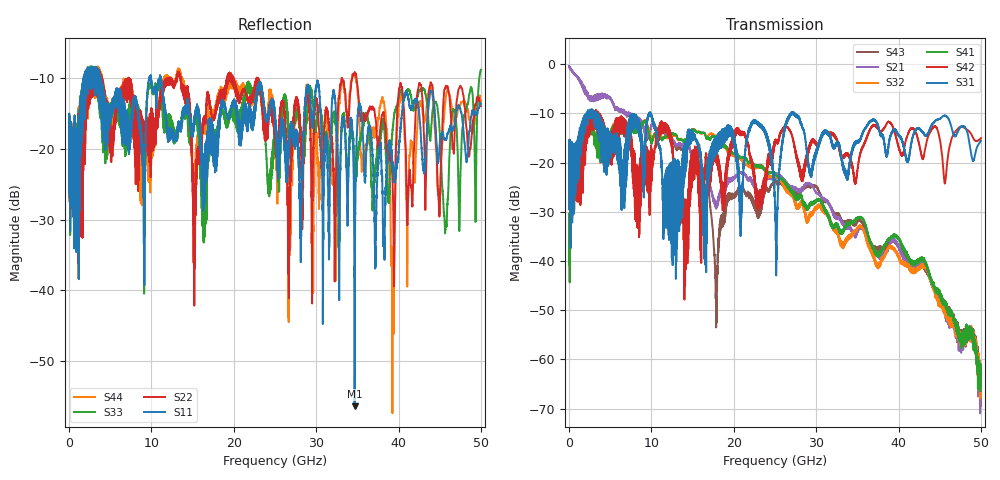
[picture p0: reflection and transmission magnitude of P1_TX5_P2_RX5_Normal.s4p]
!Keysight Technologies,N5225A,MY51441389,A.10.49.11
!Date: Monday, July 08, 2019 11:26:59
!Correction: S11(Full 4 Port(1,2,3,4))
!S12(Full 4 Port(1,2,3,4))
!S13(Full 4 Port(1,2,3,4))
!S14(Full 4 Port(1,2,3,4))
!S21(Full 4 Port(1,2,3,4))
!S22(Full 4 Port(1,2,3,4))
!S23(Full 4 Port(1,2,3,4))
!S24(Full 4 Port(1,2,3,4))
!S31(Full 4 Port(1,2,3,4))
!S32(Full 4 Port(1,2,3,4))
!S33(Full 4 Port(1,2,3,4))
!S34(Full 4 Port(1,2,3,4))
!S41(Full 4 Port(1,2,3,4))
!S42(Full 4 Port(1,2,3,4))
!S43(Full 4 Port(1,2,3,4))
!S44(Full 4 Port(1,2,3,4))
!S4P File: Measurements: <S11,S12,S13,S14>,
!<S21,S22,S23,S24>,
!<S31,S32,S33,S34>,
!<S41,S42,S43,S44>:
# Hz S  dB  R 50
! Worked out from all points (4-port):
!   5000 points, 10 MHz to 50 GHz, reference 50 ohm
!   strongest paths, dB at 10 MHz, 12.51 GHz, 25.01 GHz, 37.51 GHz, 50 GHz:
!     S31: -19.1, -20.2, -28.0, -12.5, -15.6
!     S42: -19.1, -17.4, -16.2, -13.1, -15.0
!     S41: -33.1, -14.0, -22.2, -38.6, -63.7
!     S32: -33.0, -14.3, -22.7, -41.1, -65.6
!     S21: -0.4, -15.1, -22.7, -38.8, -61.4
!     S43: -0.4, -15.6, -23.6, -37.4, -69.5
!   lowest |S11| = -56.4 dB at 34.67 GHz (marker M1), VSWR 1.00, Z = 49.9 + j0.0937 ohm
!   |S11| at or under -10 dB: start of sweep to 1.789 GHz; 3.811 GHz to 9.748 GHz (5.937 GHz wide, 87.6 % of centre); 11.15 GHz to end of sweep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
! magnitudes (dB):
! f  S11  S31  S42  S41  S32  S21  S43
! 10 MHz  -17.6  -19.1  -19.1  -33.1  -33.0  -0.4  -0.4
! 17.83 GHz  -19.8  -15.4  -18.3  -15.0  -14.8  -29.3  -46.8
! 34.67 GHz  -56.4  -16.5  -24.0  -31.9  -34.0  -34.9  -32.6
! 39.28 GHz  -22.8  -13.6  -12.6  -35.1  -37.5  -36.0  -36.1
! 40.25 GHz  -16.9  -15.0  -17.9  -36.1  -40.0  -38.1  -38.0
! 45.7 GHz  -18.8  -10.5  -23.7  -49.2  -51.4  -50.9  -49.4
! 50 GHz  -13.7  -15.6  -15.0  -63.7  -65.6  -61.4  -69.5
